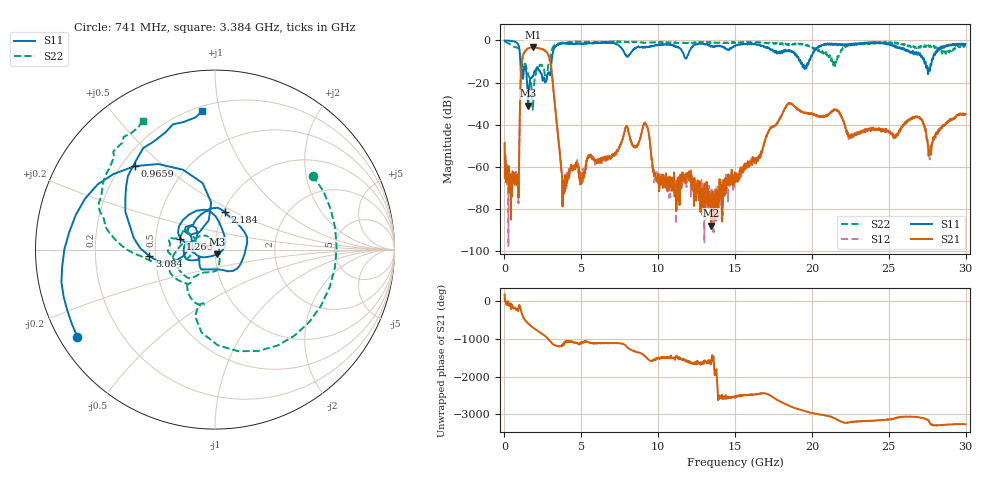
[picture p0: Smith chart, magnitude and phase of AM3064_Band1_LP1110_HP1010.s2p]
# Hz S DB R 50.0
!freq dBS11 angS11 dBS21 angS21 dBS12 angS12 dBS22 angS22
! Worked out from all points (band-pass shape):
!   1600 points, 10 MHz to 29.98 GHz, reference 50 ohm
!   highest |S21| = -3.29 dB at 1.884 GHz (marker M1); lowest = -87.8 dB at 13.43 GHz (marker M2)
!   |S21| within 3 dB of the highest: 1.25 GHz to 2.81 GHz (1.559 GHz wide, 76.8 % of centre)
!   lowest |S11| = -30.9 dB at 1.547 GHz (marker M3), VSWR 1.06, Z = 50.9 - j2.72 ohm
!   |S11| at or under -10 dB: 1.031 GHz to 3.063 GHz (2.031 GHz wide, 99.2 % of centre); 19.25 GHz to 19.8 GHz (555.2 MHz wide, 2.84 % of centre); 27.3 GHz to 27.79 GHz (487.7 MHz wide, 1.77 % of centre)
!   |S22| runs from -32.9 to -0.3 dB; largest |S21 - S12| = 0.0089
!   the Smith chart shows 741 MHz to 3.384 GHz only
!   S11 on the Smith chart (normalised r, x): 741 MHz: 0.05, -0.29; 965.9 MHz: 0.25, +0.40; 1.266 GHz: 0.67, +0.09; 2.184 GHz: 1.01, +0.45; 3.084 GHz: 0.46, -0.04; 3.384 GHz: 0.23, +0.88
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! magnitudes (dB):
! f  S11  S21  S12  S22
! 10 MHz  -0.1  -48.6  -56.9  -0.3
! 741 MHz  -0.8  -64.1  -66.9  -3.3
! 965.9 MHz  -3.8  -48.9  -50.0  -4.7
! 1.135 GHz  -13.7  -10.0  -10.0  -10.4
! 1.266 GHz  -13.9  -6.1  -6.0  -12.1
! 1.547 GHz  -30.9  -3.8  -3.7  -16.2
! 1.884 GHz  -16.7  -3.3  -3.3  -26.7
! 2.184 GHz  -13.2  -3.7  -3.7  -12.8
! 3.084 GHz  -8.7  -15.7  -15.7  -4.5
! 3.384 GHz  -2.2  -38.2  -38.1  -1.7
! 3.871 GHz  -1.3  -71.8  -67.3  -1.1
! 5.015 GHz  -1.4  -67.8  -65.5  -0.6
! 9.157 GHz  -3.3  -39.3  -39.0  -1.2
! 10 GHz  -2.2  -64.7  -67.9  -0.9
! 13.43 GHz  -2.7  -87.8  -78.2  -1.2
! 15 GHz  -2.5  -67.5  -65.2  -1.3
! 18.45 GHz  -5.1  -30.1  -30.0  -2.1
! 19.99 GHz  -7.6  -34.8  -34.9  -3.1
! 25 GHz  -1.5  -42.8  -43.6  -1.1
! 26.94 GHz  -6.2  -36.4  -36.4  -3.4
! 27.68 GHz  -13.5  -53.3  -54.1  -2.6
! 29.98 GHz  -1.8  -35.1  -35.4  -2.8
